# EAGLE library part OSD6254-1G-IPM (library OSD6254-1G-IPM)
System-On-Modules - SOM System-in-Package: Texas Instruments AM6254 ARM Quad Cortex A53 Processor, 1GB DDR4, Passives - 9mm X 14mm 500 Ball BGA - -40C to 85C Source: Datasheet
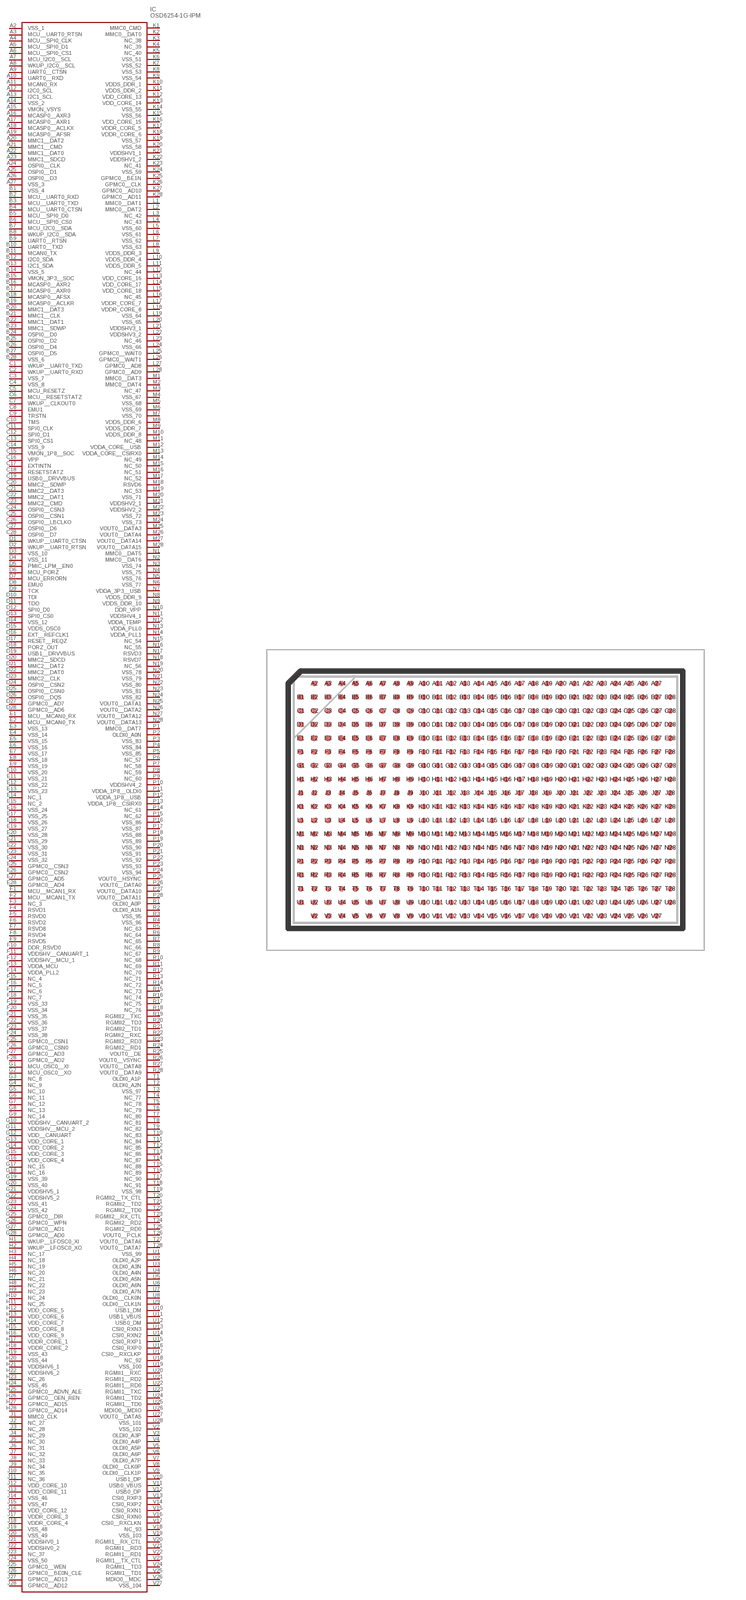
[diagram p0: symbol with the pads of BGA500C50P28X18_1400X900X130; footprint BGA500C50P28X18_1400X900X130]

Designator prefix IC

## OSD6254-1G-IPM (Description: System-On-Modules - SOM System-in-Package: Texas Instruments AM6254 ARM Quad Cortex A53 Processor, 1GB DDR4, Passives - 9mm X 14mm 500 Ball BGA - -40C to 85C; Height: 1.3mm; Manufacturer_Name: Octavo Systems; Manufacturer_Part_Number: OSD6254-1G-IPM)  [BGA500C50P28X18_1400X900X130]
A2  VSS_1
A3  MCU__UART0_RTSN
A4  MCU__SPI0_CLK
A5  MCU__SPI0_D1
A6  MCU__SPI0_CS1
A7  MCU_I2C0__SCL
A8  WKUP_I2C0__SCL
A9  UART0__CTSN
A10  UART0__RXD
A11  MCAN0_RX
A12  I2C0_SCL
A13  I2C1_SCL
A14  VSS_2
A15  VMON_VSYS
A16  MCASP0__AXR3
A17  MCASP0__AXR1
A18  MCASP0__ACLKX
A19  MCASP0__AFSR
A20  MMC1__DAT2
A21  MMC1__CMD
A22  MMC1__DAT0
A23  MMC1__SDCD
A24  OSPI0__CLK
A25  OSPI0__D1
A26  OSPI0__D3
A27  VSS_3
B1  VSS_4
B2  MCU__UART0_RXD
B3  MCU__UART0_TXD
B4  MCU__UART0_CTSN
B5  MCU__SPI0_D0
B6  MCU__SPI0_CS0
B7  MCU_I2C0__SDA
B8  WKUP_I2C0__SDA
B9  UART0__RTSN
B10  UART0__TXD
B11  MCAN0_TX
B12  I2C0_SDA
B13  I2C1_SDA
B14  VSS_5
B15  VMON_3P3__SOC
B16  MCASP0__AXR2
B17  MCASP0__AXR0
B18  MCASP0__AFSX
B19  MCASP0__ACLKR
B20  MMC1__DAT3
B21  MMC1__CLK
B22  MMC1__DAT1
B23  MMC1__SDWP
B24  OSPI0__D0
B25  OSPI0__D2
B26  OSPI0__D4
B27  OSPI0__D5
B28  VSS_6
C1  WKUP__UART0_TXD
C2  WKUP__UART0_RXD
C3  VSS_7
C4  VSS_8
C5  MCU_RESETZ
C6  MCU__RESETSTATZ
C7  WKUP__CLKOUT0
C8  EMU1
C9  TRSTN
C10  TMS
C11  SPI0_CLK
C12  SPI0_D1
C13  SPI0_CS1
C14  VSS_9
C15  VMON_1P8__SOC
C16  VPP
C17  EXTINTN
C18  RESETSTATZ
C19  USB0__DRVVBUS
C20  MMC2__SDWP
C21  MMC2__DAT3
C22  MMC2__DAT1
C23  MMC2__CMD
C24  OSPI0__CSN3
C25  OSPI0__CSN1
C26  OSPI0__LBCLKO
C27  OSPI0__D6
C28  OSPI0__D7
D1  WKUP__UART0_CTSN
D2  WKUP__UART0_RTSN
D3  VSS_10
D4  VSS_11
D5  PMIC_LPM__EN0
D6  MCU_PORZ
D7  MCU_ERRORN
D8  EMU0
D9  TCK
D10  TDI
D11  TDO
D12  SPI0_D0
D13  SPI0_CS0
D14  VSS_12
D15  VDDS_OSC0
D16  EXT__REFCLK1
D17  RESET__REQZ
D18  PORZ_OUT
D19  USB1__DRVVBUS
D20  MMC2__SDCD
D21  MMC2__DAT2
D22  MMC2__DAT0
D23  MMC2__CLK
D24  OSPI0__CSN2
D25  OSPI0__CSN0
D26  OSPI0__DQS
D27  GPMC0__AD7
D28  GPMC0__AD6
E1  MCU__MCAN0_RX
E2  MCU__MCAN0_TX
E3  VSS_13
E4  VSS_14
E5  VSS_15
E6  VSS_16
E7  VSS_17
E8  VSS_18
E9  VSS_19
E10  VSS_20
E11  VSS_21
E12  VSS_22
E13  VSS_23
E14  NC_1
E15  NC_2
E16  VSS_24
E17  VSS_25
E18  VSS_26
E19  VSS_27
E20  VSS_28
E21  VSS_29
E22  VSS_30
E23  VSS_31
E24  VSS_32
E25  GPMC0__CSN3
E26  GPMC0__CSN2
E27  GPMC0__AD5
E28  GPMC0__AD4
F1  MCU__MCAN1_RX
F2  MCU__MCAN1_TX
F3  NC_3
F4  RSVD1
F5  RSVD0
F6  RSVD2
F7  RSVD8
F8  RSVD4
F9  RSVD5
F10  DDR_RSVD0
F11  VDDSHV__CANUART_1
F12  VDDSHV__MCU_1
F13  VDDA_MCU
F14  VDDA_PLL2
F15  NC_4
F16  NC_5
F17  NC_6
F18  NC_7
F19  VSS_33
F20  VSS_34
F21  VSS_35
F22  VSS_36
F23  VSS_37
F24  VSS_38
F25  GPMC0__CSN1
F26  GPMC0__CSN0
F27  GPMC0__AD3
F28  GPMC0__AD2
G1  MCU_OSC0__XI
G2  MCU_OSC0__XO
G3  NC_8
G4  NC_9
G5  NC_10
G6  NC_11
G7  NC_12
G8  NC_13
G9  NC_14
G10  VDDSHV__CANUART_2
G11  VDDSHV__MCU_2
G12  VDD__CANUART
G13  VDD_CORE_1
G14  VDD_CORE_2
G15  VDD_CORE_3
G16  VDD_CORE_4
G17  NC_15
G18  NC_16
G19  VSS_39
G20  VSS_40
G21  VDDSHV5_1
G22  VDDSHV5_2
G23  VSS_41
G24  VSS_42
G25  GPMC0__DIR
G26  GPMC0__WPN
G27  GPMC0__AD1
G28  GPMC0__AD0
H1  WKUP__LFOSC0_XI
H2  WKUP__LFOSC0_XO
H3  NC_17
H4  NC_18
H5  NC_19
H6  NC_20
H7  NC_21
H8  NC_22
H9  NC_23
H10  NC_24
H11  NC_25
H12  VDD_CORE_5
H13  VDD_CORE_6
H14  VDD_CORE_7
H15  VDD_CORE_8
H16  VDD_CORE_9
H17  VDDR_CORE_1
H18  VDDR_CORE_2
H19  VSS_43
H20  VSS_44
H21  VDDSHV6_1
H22  VDDSHV6_2
H23  NC_26
H24  VSS_45
H25  GPMC0__ADVN_ALE
H26  GPMC0__OEN_REN
H27  GPMC0__AD15
H28  GPMC0__AD14
J1  MMC0_CLK
J2  NC_27
J3  NC_28
J4  NC_29
J5  NC_30
J6  NC_31
J7  NC_32
J8  NC_33
J9  NC_34
J10  NC_35
J11  NC_36
J12  VDD_CORE_10
J13  VDD_CORE_11
J14  VSS_46
J15  VSS_47
J16  VDD_CORE_12
J17  VDDR_CORE_3
J18  VDDR_CORE_4
J19  VSS_48
J20  VSS_49
J21  VDDSHV0_1
J22  VDDSHV0_2
J23  NC_37
J24  VSS_50
J25  GPMC0__WEN
J26  GPMC0__BE0N_CLE
J27  GPMC0__AD13
J28  GPMC0__AD12
K1  MMC0_CMD
K2  MMC0__DAT0
K3  NC_38
K4  NC_39
K5  NC_40
K6  VSS_51
K7  VSS_52
K8  VSS_53
K9  VSS_54
K10  VDDS_DDR_1
K11  VDDS_DDR_2
K12  VDD_CORE_13
K13  VDD_CORE_14
K14  VSS_55
K15  VSS_56
K16  VDD_CORE_15
K17  VDDR_CORE_5
K18  VDDR_CORE_6
K19  VSS_57
K20  VSS_58
K21  VDDSHV1_1
K22  VDDSHV1_2
K23  NC_41
K24  VSS_59
K25  GPMC0__BE1N
K26  GPMC0__CLK
K27  GPMC0__AD10
K28  GPMC0__AD11
L1  MMC0__DAT1
L2  MMC0__DAT2
L3  NC_42
L4  NC_43
L5  VSS_60
L6  VSS_61
L7  VSS_62
L8  VSS_63
L9  VDDS_DDR_3
L10  VDDS_DDR_4
L11  VDDS_DDR_5
L12  NC_44
L13  VDD_CORE_16
L14  VDD_CORE_17
L15  VDD_CORE_18
L16  NC_45
L17  VDDR_CORE_7
L18  VDDR_CORE_8
L19  VSS_64
L20  VSS_65
L21  VDDSHV3_1
L22  VDDSHV3_2
L23  NC_46
L24  VSS_66
L25  GPMC0__WAIT0
L26  GPMC0__WAIT1
L27  GPMC0__AD8
L28  GPMC0__AD9
M1  MMC0__DAT3
M2  MMC0__DAT4
M3  NC_47
M4  VSS_67
M5  VSS_68
M6  VSS_69
M7  VSS_70
M8  VDDS_DDR_6
M9  VDDS_DDR_7
M10  VDDS_DDR_8
M11  NC_48
M12  VDDA_CORE__USB
M13  VDDA_CORE__CSIRX0
M14  NC_49
M15  NC_50
M16  NC_51
M17  NC_52
M18  RSVD6
M19  NC_53
M20  VSS_71
M21  VDDSHV2_1
M22  VDDSHV2_2
M23  VSS_72
M24  VSS_73
M25  VOUT0__DATA3
M26  VOUT0__DATA4
M27  VOUT0__DATA14
M28  VOUT0__DATA15
N1  MMC0__DAT5
N2  MMC0__DAT6
N3  VSS_74
N4  VSS_75
N5  VSS_76
N6  VSS_77
N7  VDDA_3P3__USB
N8  VDDS_DDR_9
N9  VDDS_DDR_10
N10  DDR_VPP
N11  VDDSHV4_1
N12  VDDA_TEMP
N13  VDDA_PLL0
N14  VDDA_PLL1
N15  NC_54
N16  NC_55
N17  RSVD3
N18  RSVD7
N19  NC_56
N20  VSS_78
N21  VSS_79
N22  VSS_80
N23  VSS_81
N24  VSS_82
N25  VOUT0__DATA1
N26  VOUT0__DATA2
N27  VOUT0__DATA12
N28  VOUT0__DATA13
P1  MMC0__DAT7
P2  OLDI0_A0N
P3  VSS_83
P4  VSS_84
P5  VSS_85
P6  NC_57
P7  NC_58
P8  NC_59
P9  NC_60
P10  VDDSHV4_2
P11  VDDA_1P8__OLDI0
P12  VDDA_1P8__USB
P13  VDDA_1P8__CSIRX0
P14  NC_61
P15  NC_62
P16  VSS_86
P17  VSS_87
P18  VSS_88
P19  VSS_89
P20  VSS_90
P21  VSS_91
P22  VSS_92
P23  VSS_93
P24  VSS_94
P25  VOUT0__HSYNC
P26  VOUT0__DATA0
P27  VOUT0__DATA10
P28  VOUT0__DATA11
R1  OLDI0_A0P
R2  OLDI0_A1N
R3  VSS_95
R4  VSS_96
R5  NC_63
R6  NC_64
R7  NC_65
R8  NC_66
R9  NC_67
R10  NC_68
R11  NC_69
R12  NC_70
R13  NC_71
R14  NC_72
R15  NC_73
R16  NC_74
R17  NC_75
R18  NC_76
R19  RGMII2__TXC
R20  RGMII2__TD3
R21  RGMII2__TD1
R22  RGMII2__RXC
R23  RGMII2__RD3
R24  RGMII2__RD1
R25  VOUT0__DE
R26  VOUT0__VSYNC
R27  VOUT0__DATA8
R28  VOUT0__DATA9
T1  OLDI0_A1P
T2  OLDI0_A2N
T3  VSS_97
T4  NC_77
T5  NC_78
T6  NC_79
T7  NC_80
T8  NC_81
T9  NC_82
T10  NC_83
T11  NC_84
T12  NC_85
T13  NC_86
T14  NC_87
T15  NC_88
T16  NC_89
T17  NC_90
T18  NC_91
T19  VSS_98
T20  RGMII2__TX_CTL
T21  RGMII2__TD2
T22  RGMII2__TD0
T23  RGMII2__RX_CTL
T24  RGMII2__RD2
T25  RGMII2__RD0
T26  VOUT0__PCLK
T27  VOUT0__DATA6
T28  VOUT0__DATA7
U1  VSS_99
U2  OLDI0_A2P
U3  OLDI0_A3N
U4  OLDI0_A4N
U5  OLDI0_A5N
U6  OLDI0_A6N
U7  OLDI0_A7N
U8  OLDI0__CLK0N
U9  OLDI0__CLK1N
U10  USB1_DM
U11  USB1_VBUS
U12  USB0_DM
U13  CSI0_RXN3
U14  CSI0_RXN2
U15  CSI0_RXP1
U16  CSI0_RXP0
U17  CSI0__RXCLKP
U18  NC_92
U19  VSS_100
U20  RGMII1__RXC
U21  RGMII1__RD2
U22  RGMII1__RD0
U23  RGMII1__TXC
U24  RGMII1__TD2
U25  RGMII1__TD0
U26  MDIO0__MDIO
U27  VOUT0__DATA5
U28  VSS_101
V2  VSS_102
V3  OLDI0_A3P
V4  OLDI0_A4P
V5  OLDI0_A5P
V6  OLDI0_A6P
V7  OLDI0_A7P
V8  OLDI0__CLK0P
V9  OLDI0__CLK1P
V10  USB1_DP
V11  USB0_VBUS
V12  USB0_DP
V13  CSI0_RXP3
V14  CSI0_RXP2
V15  CSI0_RXN1
V16  CSI0_RXN0
V17  CSI0__RXCLKN
V18  NC_93
V19  VSS_103
V20  RGMII1__RX_CTL
V21  RGMII1__RD3
V22  RGMII1__RD1
V23  RGMII1__TX_CTL
V24  RGMII1__TD3
V25  RGMII1__TD1
V26  MDIO0__MDC
V27  VSS_104

## Footprint BGA500C50P28X18_1400X900X130 (pad centres in mm)
500-LFBGA (9x14)
smd 0.2 x 0.2: A2 -6.25,4.25; A3 -5.75,4.25; A4 -5.25,4.25; A5 -4.75,4.25; A6 -4.25,4.25; A7 -3.75,4.25; A8 -3.25,4.25; A9 -2.75,4.25; A10 -2.25,4.25; A11 -1.75,4.25; A12 -1.25,4.25; A13 -0.75,4.25; A14 -0.25,4.25; A15 0.25,4.25; A16 0.75,4.25; A17 1.25,4.25; A18 1.75,4.25; A19 2.25,4.25; A20 2.75,4.25; A21 3.25,4.25; A22 3.75,4.25; A23 4.25,4.25; A24 4.75,4.25; A25 5.25,4.25; A26 5.75,4.25; A27 6.25,4.25; B1 -6.75,3.75; B2 -6.25,3.75; B3 -5.75,3.75; B4 -5.25,3.75; B5 -4.75,3.75; B6 -4.25,3.75; B7 -3.75,3.75; B8 -3.25,3.75; B9 -2.75,3.75; B10 -2.25,3.75; B11 -1.75,3.75; B12 -1.25,3.75; B13 -0.75,3.75; B14 -0.25,3.75; B15 0.25,3.75; B16 0.75,3.75; B17 1.25,3.75; B18 1.75,3.75; B19 2.25,3.75; B20 2.75,3.75; B21 3.25,3.75; B22 3.75,3.75; B23 4.25,3.75; B24 4.75,3.75; B25 5.25,3.75; B26 5.75,3.75; B27 6.25,3.75; B28 6.75,3.75; C1 -6.75,3.25; C2 -6.25,3.25; C3 -5.75,3.25; C4 -5.25,3.25; C5 -4.75,3.25; C6 -4.25,3.25; C7 -3.75,3.25; C8 -3.25,3.25; C9 -2.75,3.25; C10 -2.25,3.25; C11 -1.75,3.25; C12 -1.25,3.25; C13 -0.75,3.25; C14 -0.25,3.25; C15 0.25,3.25; C16 0.75,3.25; C17 1.25,3.25; C18 1.75,3.25; C19 2.25,3.25; C20 2.75,3.25; C21 3.25,3.25; C22 3.75,3.25; C23 4.25,3.25; C24 4.75,3.25; C25 5.25,3.25; C26 5.75,3.25; C27 6.25,3.25; C28 6.75,3.25; D1 -6.75,2.75; D2 -6.25,2.75; D3 -5.75,2.75; D4 -5.25,2.75; D5 -4.75,2.75; D6 -4.25,2.75; D7 -3.75,2.75; D8 -3.25,2.75; D9 -2.75,2.75; D10 -2.25,2.75; D11 -1.75,2.75; D12 -1.25,2.75; D13 -0.75,2.75; D14 -0.25,2.75; D15 0.25,2.75; D16 0.75,2.75; D17 1.25,2.75; D18 1.75,2.75; D19 2.25,2.75; D20 2.75,2.75; D21 3.25,2.75; D22 3.75,2.75; D23 4.25,2.75; D24 4.75,2.75; D25 5.25,2.75; D26 5.75,2.75; D27 6.25,2.75; D28 6.75,2.75; E1 -6.75,2.25; E2 -6.25,2.25; E3 -5.75,2.25; E4 -5.25,2.25; E5 -4.75,2.25; E6 -4.25,2.25; E7 -3.75,2.25; E8 -3.25,2.25; E9 -2.75,2.25; E10 -2.25,2.25; E11 -1.75,2.25; E12 -1.25,2.25; E13 -0.75,2.25; E14 -0.25,2.25; E15 0.25,2.25; E16 0.75,2.25; E17 1.25,2.25; E18 1.75,2.25; E19 2.25,2.25; E20 2.75,2.25; E21 3.25,2.25; E22 3.75,2.25; E23 4.25,2.25; E24 4.75,2.25; E25 5.25,2.25; E26 5.75,2.25; E27 6.25,2.25; E28 6.75,2.25; F1 -6.75,1.75; F2 -6.25,1.75; F3 -5.75,1.75; F4 -5.25,1.75; F5 -4.75,1.75; F6 -4.25,1.75; F7 -3.75,1.75; F8 -3.25,1.75; F9 -2.75,1.75; F10 -2.25,1.75; F11 -1.75,1.75; F12 -1.25,1.75; F13 -0.75,1.75; F14 -0.25,1.75; F15 0.25,1.75; F16 0.75,1.75; F17 1.25,1.75; F18 1.75,1.75; F19 2.25,1.75; F20 2.75,1.75; F21 3.25,1.75; F22 3.75,1.75; F23 4.25,1.75; F24 4.75,1.75; F25 5.25,1.75; F26 5.75,1.75; F27 6.25,1.75; F28 6.75,1.75; G1 -6.75,1.25; G2 -6.25,1.25; G3 -5.75,1.25; G4 -5.25,1.25; G5 -4.75,1.25; G6 -4.25,1.25; G7 -3.75,1.25; G8 -3.25,1.25; G9 -2.75,1.25; G10 -2.25,1.25; G11 -1.75,1.25; G12 -1.25,1.25; G13 -0.75,1.25; G14 -0.25,1.25; G15 0.25,1.25; G16 0.75,1.25; G17 1.25,1.25; G18 1.75,1.25; G19 2.25,1.25; G20 2.75,1.25; G21 3.25,1.25; G22 3.75,1.25; G23 4.25,1.25; G24 4.75,1.25; G25 5.25,1.25; G26 5.75,1.25; G27 6.25,1.25; G28 6.75,1.25; H1 -6.75,0.75; H2 -6.25,0.75; H3 -5.75,0.75; H4 -5.25,0.75; H5 -4.75,0.75; H6 -4.25,0.75; H7 -3.75,0.75; H8 -3.25,0.75; H9 -2.75,0.75; H10 -2.25,0.75; H11 -1.75,0.75; H12 -1.25,0.75; H13 -0.75,0.75; H14 -0.25,0.75; H15 0.25,0.75; H16 0.75,0.75; H17 1.25,0.75; H18 1.75,0.75; H19 2.25,0.75; H20 2.75,0.75; H21 3.25,0.75; H22 3.75,0.75; H23 4.25,0.75; H24 4.75,0.75; H25 5.25,0.75; H26 5.75,0.75; H27 6.25,0.75; H28 6.75,0.75; J1 -6.75,0.25; J2 -6.25,0.25; J3 -5.75,0.25; J4 -5.25,0.25; J5 -4.75,0.25; J6 -4.25,0.25; J7 -3.75,0.25; J8 -3.25,0.25; J9 -2.75,0.25; J10 -2.25,0.25; J11 -1.75,0.25; J12 -1.25,0.25; J13 -0.75,0.25; J14 -0.25,0.25; J15 0.25,0.25; J16 0.75,0.25; J17 1.25,0.25; J18 1.75,0.25; J19 2.25,0.25; J20 2.75,0.25; J21 3.25,0.25; J22 3.75,0.25; J23 4.25,0.25; J24 4.75,0.25; J25 5.25,0.25; J26 5.75,0.25; J27 6.25,0.25; J28 6.75,0.25; K1 -6.75,-0.25; K2 -6.25,-0.25; K3 -5.75,-0.25; K4 -5.25,-0.25; K5 -4.75,-0.25; K6 -4.25,-0.25; K7 -3.75,-0.25; K8 -3.25,-0.25; K9 -2.75,-0.25; K10 -2.25,-0.25; K11 -1.75,-0.25; K12 -1.25,-0.25; K13 -0.75,-0.25; K14 -0.25,-0.25; K15 0.25,-0.25; K16 0.75,-0.25; K17 1.25,-0.25; K18 1.75,-0.25; K19 2.25,-0.25; K20 2.75,-0.25; K21 3.25,-0.25; K22 3.75,-0.25; K23 4.25,-0.25; K24 4.75,-0.25; K25 5.25,-0.25; K26 5.75,-0.25; K27 6.25,-0.25; K28 6.75,-0.25; L1 -6.75,-0.75; L2 -6.25,-0.75; L3 -5.75,-0.75; L4 -5.25,-0.75; L5 -4.75,-0.75; L6 -4.25,-0.75; L7 -3.75,-0.75; L8 -3.25,-0.75; L9 -2.75,-0.75; L10 -2.25,-0.75; L11 -1.75,-0.75; L12 -1.25,-0.75; L13 -0.75,-0.75; L14 -0.25,-0.75; L15 0.25,-0.75; L16 0.75,-0.75; L17 1.25,-0.75; L18 1.75,-0.75; L19 2.25,-0.75; L20 2.75,-0.75; L21 3.25,-0.75; L22 3.75,-0.75; L23 4.25,-0.75; L24 4.75,-0.75; L25 5.25,-0.75; L26 5.75,-0.75; L27 6.25,-0.75; L28 6.75,-0.75; M1 -6.75,-1.25; M2 -6.25,-1.25; M3 -5.75,-1.25; M4 -5.25,-1.25; M5 -4.75,-1.25; M6 -4.25,-1.25; M7 -3.75,-1.25; M8 -3.25,-1.25; M9 -2.75,-1.25; M10 -2.25,-1.25; M11 -1.75,-1.25; M12 -1.25,-1.25; M13 -0.75,-1.25; M14 -0.25,-1.25; M15 0.25,-1.25; M16 0.75,-1.25; M17 1.25,-1.25; M18 1.75,-1.25; M19 2.25,-1.25; M20 2.75,-1.25; M21 3.25,-1.25; M22 3.75,-1.25; M23 4.25,-1.25; M24 4.75,-1.25; M25 5.25,-1.25; M26 5.75,-1.25; M27 6.25,-1.25; M28 6.75,-1.25; N1 -6.75,-1.75; N2 -6.25,-1.75; N3 -5.75,-1.75; N4 -5.25,-1.75; N5 -4.75,-1.75; N6 -4.25,-1.75; N7 -3.75,-1.75; N8 -3.25,-1.75; N9 -2.75,-1.75; N10 -2.25,-1.75; N11 -1.75,-1.75; N12 -1.25,-1.75; N13 -0.75,-1.75; N14 -0.25,-1.75; N15 0.25,-1.75; N16 0.75,-1.75; N17 1.25,-1.75; N18 1.75,-1.75; N19 2.25,-1.75; N20 2.75,-1.75; N21 3.25,-1.75; N22 3.75,-1.75; N23 4.25,-1.75; N24 4.75,-1.75; N25 5.25,-1.75; N26 5.75,-1.75; N27 6.25,-1.75; N28 6.75,-1.75; P1 -6.75,-2.25; P2 -6.25,-2.25; P3 -5.75,-2.25; P4 -5.25,-2.25; P5 -4.75,-2.25; P6 -4.25,-2.25; P7 -3.75,-2.25; P8 -3.25,-2.25; P9 -2.75,-2.25; P10 -2.25,-2.25; P11 -1.75,-2.25; P12 -1.25,-2.25; P13 -0.75,-2.25; P14 -0.25,-2.25; P15 0.25,-2.25; P16 0.75,-2.25; P17 1.25,-2.25; P18 1.75,-2.25; P19 2.25,-2.25; P20 2.75,-2.25; P21 3.25,-2.25; P22 3.75,-2.25; P23 4.25,-2.25; P24 4.75,-2.25; P25 5.25,-2.25; P26 5.75,-2.25; P27 6.25,-2.25; P28 6.75,-2.25; R1 -6.75,-2.75; R2 -6.25,-2.75; R3 -5.75,-2.75; R4 -5.25,-2.75; R5 -4.75,-2.75; R6 -4.25,-2.75; R7 -3.75,-2.75; R8 -3.25,-2.75; R9 -2.75,-2.75; R10 -2.25,-2.75; R11 -1.75,-2.75; R12 -1.25,-2.75; R13 -0.75,-2.75; R14 -0.25,-2.75; R15 0.25,-2.75; R16 0.75,-2.75; R17 1.25,-2.75; R18 1.75,-2.75; R19 2.25,-2.75; R20 2.75,-2.75; R21 3.25,-2.75; R22 3.75,-2.75; R23 4.25,-2.75; R24 4.75,-2.75; R25 5.25,-2.75; R26 5.75,-2.75; R27 6.25,-2.75; R28 6.75,-2.75; T1 -6.75,-3.25; T2 -6.25,-3.25; T3 -5.75,-3.25; T4 -5.25,-3.25; T5 -4.75,-3.25; T6 -4.25,-3.25; T7 -3.75,-3.25; T8 -3.25,-3.25; T9 -2.75,-3.25; T10 -2.25,-3.25; T11 -1.75,-3.25; T12 -1.25,-3.25; T13 -0.75,-3.25; T14 -0.25,-3.25; T15 0.25,-3.25; T16 0.75,-3.25; T17 1.25,-3.25; T18 1.75,-3.25; T19 2.25,-3.25; T20 2.75,-3.25; T21 3.25,-3.25; T22 3.75,-3.25; T23 4.25,-3.25; T24 4.75,-3.25; T25 5.25,-3.25; T26 5.75,-3.25; T27 6.25,-3.25; T28 6.75,-3.25; U1 -6.75,-3.75; U2 -6.25,-3.75; U3 -5.75,-3.75; U4 -5.25,-3.75; U5 -4.75,-3.75; U6 -4.25,-3.75; U7 -3.75,-3.75; U8 -3.25,-3.75; U9 -2.75,-3.75; U10 -2.25,-3.75; U11 -1.75,-3.75; U12 -1.25,-3.75; U13 -0.75,-3.75; U14 -0.25,-3.75; U15 0.25,-3.75; U16 0.75,-3.75; U17 1.25,-3.75; U18 1.75,-3.75; U19 2.25,-3.75; U20 2.75,-3.75; U21 3.25,-3.75; U22 3.75,-3.75; U23 4.25,-3.75; U24 4.75,-3.75; U25 5.25,-3.75; U26 5.75,-3.75; U27 6.25,-3.75; U28 6.75,-3.75; V2 -6.25,-4.25; V3 -5.75,-4.25; V4 -5.25,-4.25; V5 -4.75,-4.25; V6 -4.25,-4.25; V7 -3.75,-4.25; V8 -3.25,-4.25; V9 -2.75,-4.25; V10 -2.25,-4.25; V11 -1.75,-4.25; V12 -1.25,-4.25; V13 -0.75,-4.25; V14 -0.25,-4.25; V15 0.25,-4.25; V16 0.75,-4.25; V17 1.25,-4.25; V18 1.75,-4.25; V19 2.25,-4.25; V20 2.75,-4.25; V21 3.25,-4.25; V22 3.75,-4.25; V23 4.25,-4.25; V24 4.75,-4.25; V25 5.25,-4.25; V26 5.75,-4.25; V27 6.25,-4.25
